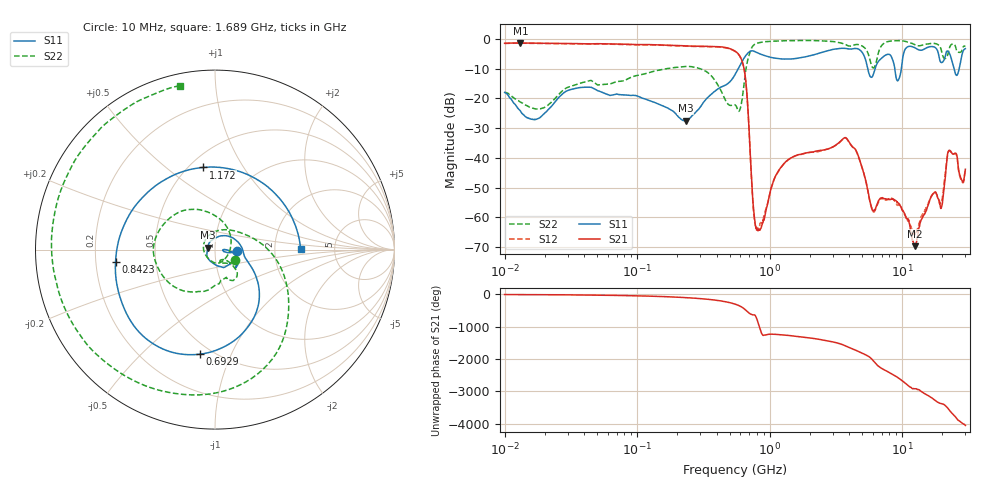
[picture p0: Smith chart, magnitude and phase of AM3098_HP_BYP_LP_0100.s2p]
!Agilent Technologies,E8364B,MY43040894,A.07.50.67
!Agilent E8364B: A.07.50.67
!Date: Wednesday, June 17, 2020 09:19:55
!Correction: S11(Full 2 Port(1,2))
!S21(Full 2 Port(1,2))
!S12(Full 2 Port(1,2))
!S22(Full 2 Port(1,2))
!S2P File: Measurements: S11, S21, S12, S22:Log Frequency Sweep
# Hz S  dB  R 50
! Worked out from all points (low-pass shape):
!   1601 points, 10 MHz to 30 GHz, reference 50 ohm
!   highest |S21| = -1.40 dB at 13.17 MHz (marker M1); lowest = -69.7 dB at 12.5 GHz (marker M2)
!   |S21| within 3 dB of the highest: start of sweep to 558 MHz
!   lowest |S11| = -27.5 dB at 232.8 MHz (marker M3), VSWR 1.09, Z = 46.1 + j1.01 ohm
!   |S11| at or under -10 dB: 5.495 GHz to 6.25 GHz (754.7 MHz wide, 12.9 % of centre); 8.795 GHz to 9.864 GHz (1.069 GHz wide, 11.5 % of centre); 24.6 GHz to 26.95 GHz (2.343 GHz wide, 9.09 % of centre)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
!   |S22| runs from -24.4 to -0.6 dB; largest |S21 - S12| = 0.014
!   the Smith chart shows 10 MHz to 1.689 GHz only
!   S11 on the Smith chart (normalised r, x): 10 MHz: 1.29, -0.01; 692.9 MHz: 0.43, -0.77; 842.3 MHz: 0.28, -0.06; 1.172 GHz: 0.58, +0.68; 1.689 GHz: 2.82, +0.02
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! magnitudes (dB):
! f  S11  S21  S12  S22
! 10 MHz  -18.0  -1.5  -1.5  -18.0
! 13.17 MHz  -24.3  -1.4  -1.5  -21.3
! 38.04 MHz  -16.3  -1.7  -1.7  -14.8
! 144.7 MHz  -21.9  -2.1  -2.1  -10.6
! 232.8 MHz  -27.5  -2.4  -2.5  -9.3
! 547.7 MHz  -12.1  -4.1  -4.2  -22.2
! 636.4 MHz  -6.7  -9.4  -9.4  -16.4
! 692.9 MHz  -4.6  -27.0  -27.2  -6.1
! 762.1 MHz  -4.2  -58.6  -59.7  -2.0
! 842.3 MHz  -5.1  -64.2  -62.5  -1.3
! 1.172 GHz  -6.7  -44.1  -44.4  -0.7
! 1.689 GHz  -6.4  -38.9  -38.9  -0.6
! 2.084 GHz  -5.6  -38.1  -38.2  -0.6
! 3.779 GHz  -3.3  -33.3  -33.4  -2.1
! 5.989 GHz  -12.5  -57.8  -57.9  -9.7
! 7.926 GHz  -5.2  -53.9  -53.8  -0.9
! 9.302 GHz  -14.1  -55.2  -56.0  -0.7
! 12.5 GHz  -3.0  -69.7  -65.7  -2.0
! 19.8 GHz  -8.0  -56.6  -54.9  -4.0
! 22.67 GHz  -4.8  -37.5  -37.7  -3.3
! 25.82 GHz  -12.3  -39.1  -39.3  -4.1
! 30 GHz  -3.3  -43.9  -44.2  -2.6
